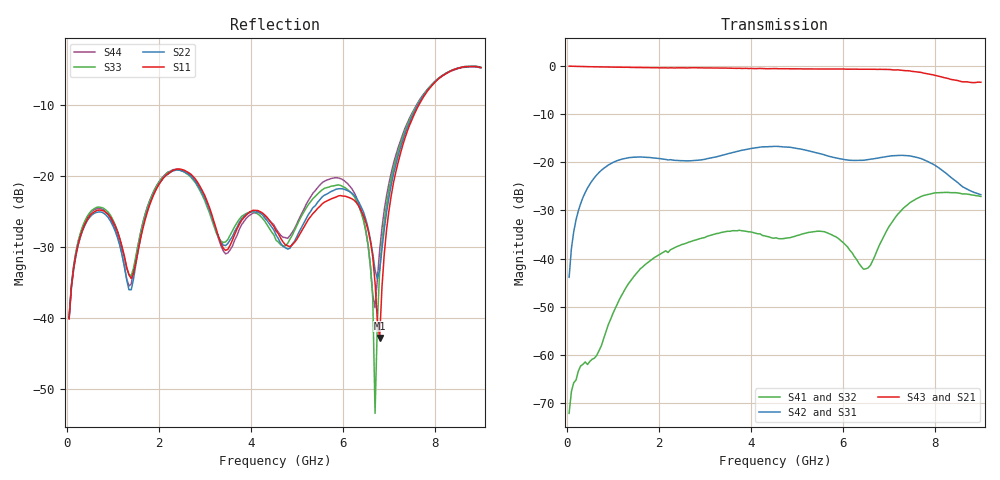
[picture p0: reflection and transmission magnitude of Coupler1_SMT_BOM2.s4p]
! Created Tue Sep 05 15:55:00 2017
# hz S ma R 50
! 4 Port Network Data from SP1.SP block
! freq  magS11  angS11  magS12  angS12  magS13  angS13  magS14  angS14
!  magS21  angS21  magS22  angS22  magS23  angS23  magS24  angS24
!  magS31  angS31  magS32  angS32  magS33  angS33  magS34  angS34
!  magS41  angS41  magS42  angS42  magS43  angS43  magS44  angS44
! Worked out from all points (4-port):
!   180 points, 50 MHz to 9 GHz, reference 50 ohm
!   strongest paths, dB at 50 MHz, 2.3 GHz, 4.55 GHz, 6.8 GHz, 9 GHz:
!     S43: -0.1, -0.4, -0.6, -0.7, -3.4
!     S21: -0.1, -0.4, -0.6, -0.7, -3.3
!     S42: -43.9, -19.6, -16.7, -19.1, -26.7
!     S31: -43.9, -19.6, -16.7, -19.1, -26.7
!     S41: -72.1, -37.9, -35.7, -37.1, -27.1
!     S32: -72.1, -37.9, -35.7, -37.1, -27.1
!   lowest |S11| = -42.8 dB at 6.8 GHz (marker M1), VSWR 1.01, Z = 50.5 - j0.504 ohm
!   |S11| at or under -10 dB: start of sweep to 7.651 GHz
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5e7  0.009842 51.0  0.994 -5.6  0.006429 82.9  0.0002128 -111.4
     0.9942 -5.6  0.00997 51.1  0.0002128 -111.4  0.006429 82.9
     0.006386 82.7  0.0002472 -122.5  0.01013 52.9  0.9952 -5.5
     0.0002472 -122.5  0.006386 82.7  0.9939 -5.6  0.01024 52.8
1.7e9  0.04896 80.5  0.9605 178.8  0.1127 -90.7  0.008612 155.3
       0.9578 178.7  0.05022 75.6  0.008614 155.3  0.1127 -90.7
       0.1129 -90.6  0.008633 155.3  0.05324 81.6  0.9612 178.9
       0.008634 155.3  0.1129 -90.6  0.9588 178.8  0.05357 77.2
3.25e9  0.04184 -81.5  0.951 14.0  0.114 104.4  0.01811 -60.6
        0.9511 13.9  0.04108 -78.2  0.0181 -60.6  0.114 104.4
        0.1137 104.5  0.01816 -61.1  0.0397 -70.3  0.9504 14.2
        0.01816 -61.1  0.1137 104.5  0.9517 14.1  0.04092 -90.9
4.2e9  0.05616 -68.8  0.9386 -87.6  0.1435 2.2  0.01782 175.5
       0.9416 -87.7  0.05476 -74.2  0.01782 175.5  0.1435 2.2
       0.1435 2.3  0.01806 175.6  0.05251 -73.6  0.9392 -87.4
       0.01805 175.6  0.1435 2.3  0.9417 -87.5  0.055 -82.0
5.05e9  0.03825 -74.9  0.9319 -179.1  0.1377 -88.7  0.01763 89.4
        0.9307 -179.3  0.04044 -77.3  0.01763 89.4  0.1377 -88.7
        0.1378 -88.7  0.01751 89.0  0.04855 -73.4  0.9302 -178.9
        0.01751 89.0  0.1378 -88.7  0.9306 -179.0  0.0499 -86.2
6.8e9  0.007232 -43.6  0.9235 -11.9  0.1115 76.5  0.01387 60.9
       0.9226 -12.0  0.02172 -171.1  0.01387 60.9  0.1115 76.5
       0.1114 76.7  0.01398 61.3  0.02155 -110.8  0.9231 -11.7
       0.01398 61.3  0.1114 76.7  0.9218 -11.9  0.03012 -127.4
9e9  0.5801 21.4  0.6797 110.1  0.04595 -109.6  0.0441 54.3
     0.6807 109.6  0.5775 26.9  0.04408 54.3  0.04595 -109.6
     0.046 -109.0  0.04407 53.9  0.583 25.3  0.678 110.0
     0.04409 53.9  0.046 -109.0  0.6766 109.4  0.5777 22.5
